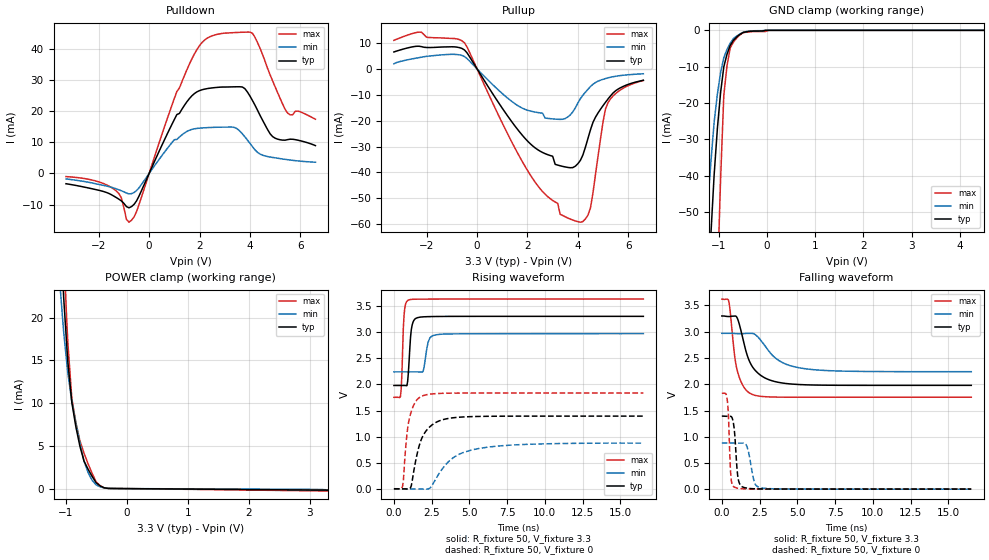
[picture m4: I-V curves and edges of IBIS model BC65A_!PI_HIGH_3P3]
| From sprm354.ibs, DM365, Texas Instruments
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|   Model Cell BC65A_!PI_HIGH_3P3
|BC1833DV65ATHYPBFZP_!PI_HIGH_3P3
[Model]   BC65A_!PI_HIGH_3P3
Model_type   I/O
Polarity   Non-Inverting
Enable   Active-Low
Vinl =  0.8V
Vinh =  2V
Cref =  15pF
Rref =  100.00M
Vref =  0V
Vmeas =  1.65
C_comp   1.512681p   1.336608p   1.607201p
[Model Spec]
Vinl   0.8V   0.8V   0.8V
Vinh   2V   2V   2V
[Temperature Range]   25   125   -40
[Voltage Range]   3.3   2.97   3.63
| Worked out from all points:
|   slope of the pulldown table from 0 to 0.495 V, typ, clamps not added: 56.1 ohm
|   slope of the pullup table from 0 to 0.495 V, typ, clamps not added: 64.3 ohm
|   GND clamp passes 1 mA (typ) near -0.55 V on its own axis
|   POWER clamp passes 1 mA (typ) near -0.53 V on its own axis
|   rising waveform, R_fixture 50, V_fixture 3.3: 20-80 % time 185ps typ, 265ps min, 141ps max; typ from 1.98 V to 3.3 V
|   rising waveform, R_fixture 50, V_fixture 0: 20-80 % time 863ps typ, 1.9ns min, 460ps max; typ from 0.005 V to 1.39 V
|   falling waveform, R_fixture 50, V_fixture 3.3: 20-80 % time 1.03ns typ, 1.61ns min, 562ps max; typ from 3.3 V to 1.98 V
|   falling waveform, R_fixture 50, V_fixture 0: 20-80 % time 212ps typ, 346ps min, 143ps max; typ from 1.39 V to 0.005 V
[POWER_clamp]
|   voltage   I(typ)   I(min)   I(max)
-3.3V     617.8mA    728.2mA    693.2mA
-1.1V     32.25mA    24.35mA    40.96mA
-1.033V   22.32mA    18.3mA     27.36mA
-966.7mV  14.93mA    13.59mA    17.23mA
-900mV    10.09mA    10.21mA    10.55mA
-833.3mV  7.224mA    7.674mA    7.713mA
-766.7mV  4.936mA    5.345mA    5.578mA
-700mV    3.224mA    3.225mA    4.147mA
-566.7mV  1.423mA    962.7uA    1.779mA
-500mV    676.6uA    428.5uA    772.2uA
-300mV    23.95uA    19.02uA    31.4uA
3.3V      -180.6uA   -149uA     -280.3uA
[Pulldown]
|   voltage   I(typ)   I(min)   I(max)
-3.3V     -3.312mA   -1.764mA   -1.021mA
-1.4V     -7.283mA   -4.687mA   -5.038mA
-1.1V     -8.831mA   -5.573mA   -7.894mA
-900mV    -10.65mA   -6.307mA   -14.75mA
-700mV    -10.64mA   -6.484mA   -15mA
1.6V      24.01mA    13.84mA    35.08mA
2.7V      27.57mA    14.8mA     44.57mA
3.7V      27.7mA     12.68mA    45.26mA
4.1V      23.38mA    8.578mA    44.92mA
4.9V      11.81mA    5.118mA    29.68mA
5.5V      10.83mA    4.397mA    19.31mA
6.6V      8.906mA    3.589mA    17.38mA
[Pullup]
|   voltage   I(typ)   I(min)   I(max)
-3.3V     6.54mA     1.969mA    11.03mA
-2.3V     8.757mA    4.357mA    14.22mA
-500mV    7.317mA    4.758mA    10.08mA
1.6V      -23.29mA   -14.09mA   -32.38mA
2.7V      -32.76mA   -19.02mA   -48.43mA
3.2V      -37.19mA   -19.48mA   -51.99mA
3.5V      -37.9mA    -19.18mA   -57.17mA
4.1V      -35.37mA   -11.52mA   -59.26mA
4.5V      -23.57mA   -6.848mA   -53.82mA
5V        -14.2mA    -4.028mA   -20.44mA
5.2V      -11.59mA   -3.459mA   -13.01mA
6.6V      -4.403mA   -1.883mA   -4.482mA
[GND_clamp]
|   voltage   I(typ)   I(min)   I(max)
-3.3V     -675.4mA   -720mA     -1.407A
-1.3V     -90.41mA   -60.43mA   -217.4mA
-1.233V   -72.69mA   -47.76mA   -178.2mA
-1.167V   -55.75mA   -35.99mA   -139.8mA
-1.1V     -39.6mA    -25.14mA   -102.2mA
-1.033V   -26.98mA   -17.51mA   -69.05mA
-966.7mV  -17.12mA   -11.63mA   -40.93mA
-900mV    -10.03mA   -7.518mA   -17.89mA
-833.3mV  -6.562mA   -5.254mA   -9.711mA
-766.7mV  -4.127mA   -3.508mA   -4.827mA
-500mV    -590uA     -557.8uA   -675.7uA
6.6V      0A         0A         0A
[Ramp]
| variable   typ   min   max
dV/dt_f  0.7923682/1.02452n   0.4387521/1.614571n   1.126032/0.5611231n
dV/dt_r  0.8364919/0.8625536n  0.5297246/1.917132n   1.099761/0.4597483n
R_load = 50
[Rising Waveform]
R_fixture = 50
V_fixture = 3.3
V_fixture_min = 2.97
V_fixture_max = 3.63
|   time   V(typ)   V(min)   V(max)
0s        1.979V     2.239V     1.753V
432ps     1.979V     2.239V     1.767V
672ps     1.979V     2.239V     3.322V
864ps     1.978V     2.239V     3.589V
1.008ns   2.46V      2.239V     3.615V
1.208ns   3.134V     2.239V     3.625V
1.708ns   3.283V     2.238V     3.628V
2.388ns   3.295V     2.891V     3.629V
2.86ns    3.297V     2.95V      3.63V
16.52ns   3.3V       2.97V      3.63V
[Rising Waveform]
R_fixture = 50
V_fixture = 0
V_fixture_min = 0
V_fixture_max = 0
|   time   V(typ)   V(min)   V(max)
0s        4.724mV    2.796mV    6.845mV
576ps     4.717mV    2.805mV    61.24mV
864ps     1.181mV    2.803mV    1.049V
1.104ns   28.78mV    2.802mV    1.439V
1.6ns     746.9mV    2.694mV    1.728V
1.932ns   1.021V     -269.8uV   1.784V
2.388ns   1.193V     17.81mV    1.813V
2.98ns    1.3V       291.9mV    1.827V
5.136ns   1.384V     746.2mV    1.835V
16.52ns   1.394V     878.4mV    1.835V
[Falling Waveform]
R_fixture = 50
V_fixture = 3.3
V_fixture_min = 2.97
V_fixture_max = 3.63
|   time   V(typ)   V(min)   V(max)
0s        3.3V       2.97V      3.622V
480ps     3.29V      2.97V      3.556V
864ps     3.299V     2.966V     2.505V
1.104ns   3.196V     2.964V     2.178V
1.656ns   2.574V     2.968V     1.875V
2.044ns   2.325V     2.968V     1.804V
2.744ns   2.138V     2.775V     1.766V
3.692ns   2.04V      2.469V     1.755V
5.136ns   1.995V     2.312V     1.753V
16.52ns   1.979V     2.239V     1.753V
[Falling Waveform]
R_fixture = 50
V_fixture = 0
V_fixture_min = 0
V_fixture_max = 0
|   time   V(typ)   V(min)   V(max)
0s        1.394V     881.4mV    1.83V
336ps     1.39V      881.3mV    1.752V
432ps     1.39V      881.3mV    1.452V
624ps     1.386V     880.8mV    173.8mV
912ps     798.7mV    879.5mV    31.93mV
1.208ns   87.77mV    879.6mV    13.58mV
1.656ns   23.36mV    820.1mV    8.035mV
2.156ns   10.45mV    136.2mV    7.098mV
2.624ns   7.258mV    27.42mV    6.914mV
16.52ns   4.716mV    2.914mV    6.828mV
